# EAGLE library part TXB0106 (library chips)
6 channel level translator
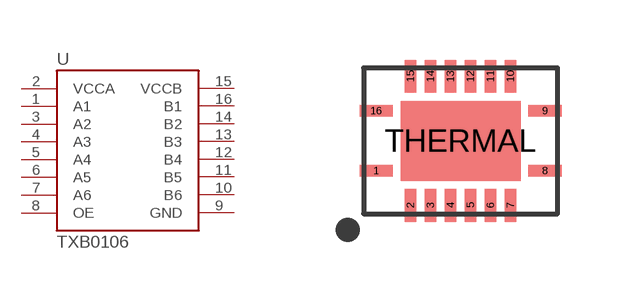
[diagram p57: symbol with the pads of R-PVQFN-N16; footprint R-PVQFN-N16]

Designator prefix -

## TXB0106 (DIGIKEY: 296-23868-2-ND)  [R-PVQFN-N16]
1  A1
2  VCCA
3  A2
4  A3
5  A4
6  A5
7  A6
8  OE
9  GND
10  B6
11  B5
12  B4
13  B3
14  B2
15  VCCB
16  B1

## Footprint R-PVQFN-N16 (pad centres in mm)
smd 0.825 x 0.28: 1 -2.112,-0.75; 8 2.112,-0.75; 9 2.112,0.75; 16 -2.112,0.75
smd 0.28 x 0.825: 2 -1.25,-1.613; 3 -0.75,-1.613; 4 -0.25,-1.613; 5 0.25,-1.613; 6 0.75,-1.613; 7 1.25,-1.613; 10 1.25,1.613; 11 0.75,1.613; 12 0.25,1.613; 13 -0.25,1.613; 14 -0.75,1.613; 15 -1.25,1.613
smd 3 x 2: THERMAL 0,0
